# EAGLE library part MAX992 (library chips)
The MAX9922/MAX9923 ultra-precision, high-side current- sense amplifiers feature ultra-low offset voltage (VOS) of 25μV (max) and laser-trimmed gain accuracy better than 0.5%. The combination of low VOS and highgain accuracy allows precise current measurements even at very small sense voltages.
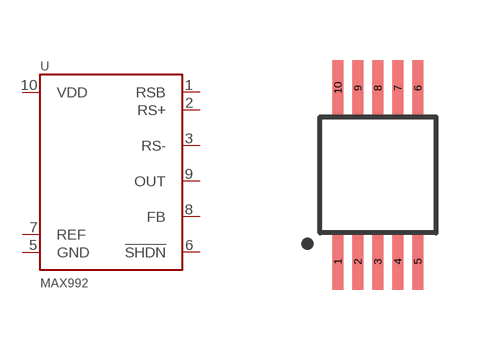
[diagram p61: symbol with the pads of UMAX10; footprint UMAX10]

Designator prefix U

## MAX9923H (DIGIKEY: MAX9923HEUB+-ND)  [UMAX10]
1  RSB
2  RS+
3  RS-
5  GND
6  !SHDN
7  REF
8  FB
9  OUT
10  VDD

## Footprint UMAX10 (pad centres in mm)
smd 0.28 x 1.4: 1 -1,-2.17; 2 -0.5,-2.17; 3 0,-2.17; 4 0.5,-2.17; 5 1,-2.17; 6 1,2.17; 7 0.5,2.17; 8 0,2.17; 9 -0.5,2.17; 10 -1,2.17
